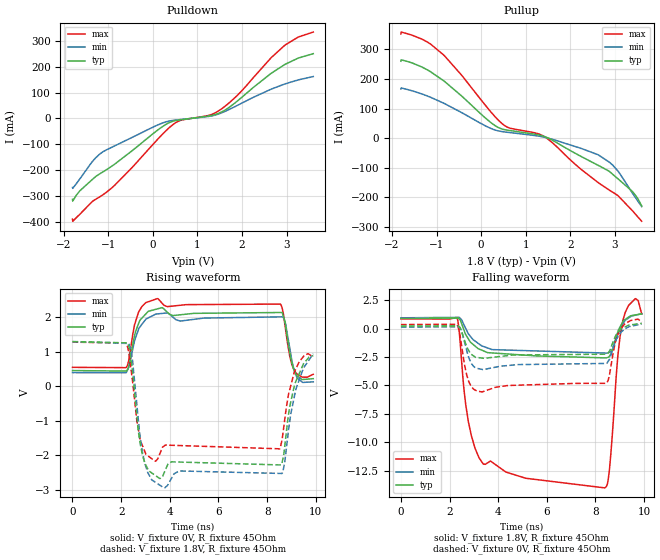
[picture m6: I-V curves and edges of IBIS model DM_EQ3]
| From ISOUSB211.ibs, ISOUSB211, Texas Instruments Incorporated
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[Model]   DM_EQ3
Model_type   Output
Polarity   Inverting
Vmeas = 0.2
Vref = 0
Cref = 15pF
Rref = 45
|   typ   min   max
C_comp   5pF   3pF   8pF
[Voltage Range]   1.8   1.71   1.89
[Temperature Range]   27   150   -40
[Pullup Reference]   1.8   1.71   1.89
[Pulldown Reference]   0   0   0
[Power Clamp Reference]   1.8   1.71   1.89
[GND Clamp Reference]   0   0   0
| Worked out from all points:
|   slope of the pulldown table from 0 to 0.27 V, typ, clamps not added: 7.95 ohm
|   slope of the pullup table from 0 to 0.27 V, typ, clamps not added: 7.94 ohm
|   falling waveform, V_fixture 1.8V, R_fixture 45Ohm: 20-80 % time 348ps typ, 328ps min, 35.7ps max; typ from 0.895 V to 1.3 V
|   rising waveform, V_fixture 0V, R_fixture 45Ohm: 20-80 % time 155ps typ, 162ps min, 102ps max; typ from 0.46 V to 0.225 V
|   rising waveform, V_fixture 1.8V, R_fixture 45Ohm: 20-80 % time 84.1ps typ, 85.9ps min, 83.5ps max; typ from 1.3 V to 0.895 V
|   falling waveform, V_fixture 0V, R_fixture 45Ohm: 20-80 % time 402ps typ, 364ps min, 86.9ps max; typ from 0.225 V to 0.46 V
[Pulldown]
|   Voltage   I(typ)   I(min)   I(max)
-1.8V     -312.3mA   -266.2mA   -388.8mA
-1.795V   -319mA     -269.8mA   -396.8mA
-1.633V   -278.9mA   -232.8mA   -369.2mA
-1.179V   -212.7mA   -136mA     -301.6mA
-865.8mV  -177.8mA   -106.8mA   -260mA
73.8mV    -49.63mA   -27.98mA   -87.09mA
538.2mV   -7.266mA   -5.626mA   -13.71mA
1.294V    10.85mA    9.019mA    13.98mA
1.521V    23.18mA    20.15mA    34.45mA
1.899V    67.71mA    50.57mA    89.7mA
2.947V    206.8mA    132.3mA    280.4mA
3.6V      250.2mA    161.9mA    333.6mA
[Pullup]
|   Voltage   I(typ)   I(min)   I(max)
-1.8V     259.8mA    166.3mA    352.1mA
-1.795V   264.8mA    169.7mA    358.5mA
-1.325V   240.1mA    149.1mA    334.3mA
-849.6mV  194.9mA    118.9mA    282mA
381.6mV   36.3mA     24.84mA    61.51mA
613.8mV   26.64mA    19.55mA    35.63mA
1.402V    6.733mA    3.773mA    6.537mA
2.612V    -90.76mA   -55.24mA   -148.5mA
2.876V    -112.3mA   -81.28mA   -175.5mA
3.065V    -136.9mA   -110.7mA   -193.6mA
3.4V      -181.3mA   -187.3mA   -246.2mA
3.6V      -228.6mA   -231.2mA   -280.5mA
[Ramp]
R_load = 45
|   typ   min   max
dV/dt_r   0.140808/1.28824e-10   0.160407/1.32946e-10   0.120509/9.80131e-11
dV/dt_f   0.243789/2.90143e-10   0.210518/2.8821e-10   0.256824/7.0026e-09
[Falling Waveform]
V_fixture = 1.8V
V_fixture_min = 1.71V
V_fixture_max = 1.89V
R_fixture = 45Ohm
C_fixture = 0F
|   Time   V(typ)   V(min)   V(max)
0s        895mV      947.6mV    856.5mV
2.304ns   936.3mV    987.1mV    973.2mV
2.766ns   -882.6mV   -441.7mV   -8.102V
3.377ns   -1.949V    -1.562V    -11.9V
8.364ns   -2.577V    -2.152V    -14.02V
8.56ns    -2.466V    -2.105V    -12.68V
8.913ns   -331.9mV   -546.4mV   -2.548V
9.11ns    546.1mV    353.8mV    547.8mV
9.632ns   1.2V       1.173V     2.627V
9.9ns     1.301V     1.298V     1.285V
[Rising Waveform]
V_fixture = 0V
V_fixture_min = 0V
V_fixture_max = 0V
R_fixture = 45Ohm
C_fixture = 0F
|   Time   V(typ)   V(min)   V(max)
0s        459.5mV    400.3mV    553.4mV
2.207ns   445.4mV    396.7mV    544.6mV
2.711ns   1.809V     1.647V     2.145V
3.487ns   2.249V     2.103V     2.548V
3.895ns   2.153V     2.133V     2.316V
8.544ns   2.144V     2.018V     2.389V
8.754ns   1.789V     1.835V     1.688V
9.093ns   506.7mV    530.2mV    498.1mV
9.461ns   200.3mV    115.4mV    269mV
9.9ns     224.9mV    133mV      352.5mV
[Rising Waveform]
V_fixture = 1.8V
V_fixture_min = 1.71V
V_fixture_max = 1.89V
R_fixture = 45Ohm
C_fixture = 0F
|   Time   V(typ)   V(min)   V(max)
0s        1.301V     1.298V     1.285V
2.316ns   1.148V     1.246V     957.1mV
2.644ns   -852.1mV   -516mV     -983.8mV
2.883ns   -2.011V    -1.926V    -1.731V
3.403ns   -2.581V    -2.779V    -2.168V
3.757ns   -2.524V    -2.942V    -1.733V
4.392ns   -2.195V    -2.452V    -1.715V
8.615ns   -2.221V    -2.526V    -1.558V
9.13ns    48.49mV    -265.8mV   427.9mV
9.9ns     895mV      947.6mV    856.5mV
[Falling Waveform]
|Gnd
V_fixture = 0V
V_fixture_min = 0V
V_fixture_max = 0V
R_fixture = 45Ohm
C_fixture = 0F
|   Time   V(typ)   V(min)   V(max)
0s        224.9mV    133mV      352.5mV
2.295ns   241.9mV    154.5mV    375.6mV
2.502ns   -315mV     -258.6mV   -1.606V
2.779ns   -1.897V    -2.469V    -4.607V
3.326ns   -2.594V    -3.585V    -5.572V
8.436ns   -2.254V    -3.069V    -4.821V
8.565ns   -2.004V    -2.736V    -4.192V
8.821ns   -669mV     -1.149V    -1.148V
9.008ns   -117.5mV   -447mV     -103.3mV
9.9ns     459.5mV    400.3mV    553.4mV
